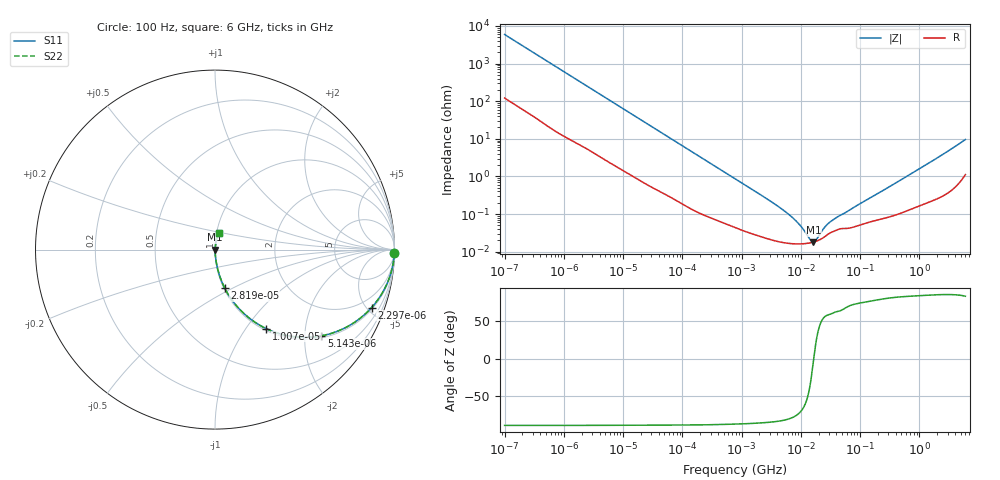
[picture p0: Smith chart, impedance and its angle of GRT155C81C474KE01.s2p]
!Murata Part Number: GRT155C81C474KE01
!These Parameters are Measured in Series Mode Connection
!Data Generated on Jun 19, 2026
!  o--ll--o
!Port1  Port2
!  o------o
!Operation Temp=25[degC], DC Bias Voltage=0[V]
!Freq. Start=100[Hz] Stop=6[GHz] 401[Steps]
# Hz S RI R 50
!Freq.(Hz) S11(Real) S11(Imag) S21(Real) S21(Imag) S12(Real) S12(Imag) S22(Real) S22(Imag)
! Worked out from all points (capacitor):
!   401 points, 100 Hz to 6 GHz, reference 50 ohm
!   read as one part in series: C = 268 nF near 109 Hz
!   lowest |Z| = 18 mohm at 16.27 MHz (marker M1)
!   series resonance near 16.51 MHz, so ESL is about 350 pH
!   S11 on the Smith chart (normalised r, x): 100 Hz: open; 2.297 kHz: 1.11, -5.35; 5.143 kHz: 1.05, -2.42; 10.07 kHz: 1.03, -1.25; 28.19 kHz: 1.01, -0.45; 6 GHz: 1.02, +0.19
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100  0.9994 -0.0169  0.000632 0.0169  0.000632 0.0169  0.9994 -0.0169
600  0.9885 -0.0977  0.0115 0.0977  0.0115 0.0977  0.9885 -0.0977
2008  0.8983 -0.2918  0.1017 0.2918  0.1017 0.2918  0.8983 -0.2918
2297  0.8723 -0.3231  0.1277 0.3231  0.1277 0.3231  0.8723 -0.3231
3437  0.7594 -0.4167  0.2406 0.4167  0.2406 0.4167  0.7594 -0.4167
5143  0.592 -0.4806  0.408 0.4806  0.408 0.4806  0.592 -0.4806
10066  0.2846 -0.4399  0.7154 0.4399  0.7154 0.4399  0.2846 -0.4399
16473  0.1342 -0.3294  0.8658 0.3294  0.8658 0.3294  0.1342 -0.3294
28191  0.0533 -0.2127  0.9467 0.2127  0.9467 0.2127  0.0533 -0.2127
40335  0.0284 -0.1536  0.9716 0.1536  0.9716 0.1536  0.0284 -0.1536
129199  0.00401 -0.0503  0.996 0.0503  0.996 0.0503  0.00401 -0.0503
774597  0.000513 -0.00869  0.9995 0.00869  0.9995 0.00869  0.000513 -0.00869
6075234  0.000169 -0.00101  0.9998 0.00101  0.9998 0.00101  0.000169 -0.00101
9506416  0.000162 -0.000501  0.9998 0.000501  0.9998 0.000501  0.000162 -0.000501
1.555665e7  0.000177 -5.14e-05  0.9998 5.14e-05  0.9998 5.14e-05  0.000177 -5.14e-05
1.626902e7  0.00018 -1.27e-05  0.9998 1.27e-05  0.9998 1.27e-05  0.00018 -1.27e-05
1.86079e7  0.000192 0.000103  0.9998 -0.000103  0.9998 -0.000103  0.000192 0.000103
2.662322e7  0.000267 0.000414  0.9997 -0.000414  0.9997 -0.000414  0.000267 0.000414
3.330331e7  0.000332 0.000578  0.9997 -0.000578  0.9997 -0.000578  0.000332 0.000578
3.124326e8  0.000868 0.00525  0.9991 -0.00525  0.9991 -0.00525  0.000868 0.00525
1.873145e9  0.00326 0.0288  0.9967 -0.0288  0.9967 -0.0288  0.00326 0.0288
6e9  0.0198 0.0924  0.9802 -0.0924  0.9802 -0.0924  0.0198 0.0924
